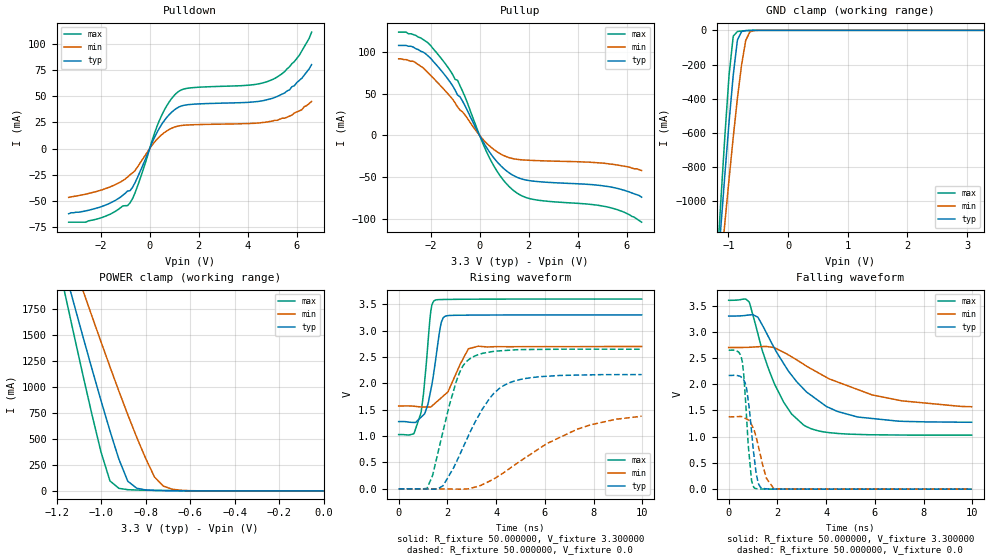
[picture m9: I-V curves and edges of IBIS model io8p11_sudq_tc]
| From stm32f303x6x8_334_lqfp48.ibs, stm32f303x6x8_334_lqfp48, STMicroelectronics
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|   Model io8p11_sudq_tc
[Model]  io8p11_sudq_tc
Model_type I/O
Polarity   Non-Inverting
Enable   Active-Low
Vinl =   0.990000V
Vinh =   2.310000V
Vmeas =  1.650000V
Cref =   30.000000pF
Rref =   100.000000M
Vref =   0.0V
C_comp   1.329900pF   1.255600pF   1.431200pF
[Temperature Range]   25.000000   0.125000k   -40.000000
[Pullup Reference]   3.300000V   2.700000V   3.600000V
[Pulldown Reference]   0.0V   0.0V   0.0V
[POWER Clamp Reference]   3.300000V   2.700000V   3.600000V
[GND Clamp Reference]   0.0V   0.0V   0.0V
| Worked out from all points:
|   slope of the pulldown table from 0 to 0.495 V, typ, clamps not added: 21.3 ohm
|   slope of the pullup table from 0 to 0.495 V, typ, clamps not added: 20.9 ohm
|   GND clamp passes 1 mA (typ) near -0.67 V on its own axis
|   POWER clamp passes 1 mA (typ) near -0.60 V on its own axis
|   rising waveform, R_fixture 50.000000, V_fixture 3.300000: 20-80 % time 415ps typ, 734ps min, 311ps max; typ from 1.27 V to 3.3 V
|   rising waveform, R_fixture 50.000000, V_fixture 0.0: 20-80 % time 1.47ns typ, 2.98ns min, 896ps max; typ from 0 V to 2.17 V
|   falling waveform, R_fixture 50.000000, V_fixture 3.300000: 20-80 % time 2.06ns typ, 3.13ns min, 1.29ns max; typ from 3.3 V to 1.27 V
|   falling waveform, R_fixture 50.000000, V_fixture 0.0: 20-80 % time 303ps typ, 447ps min, 236ps max; typ from 2.17 V to 0 V
[Pulldown]
|Voltage   I(typ)   I(min)   I(max)
-3.3V     -62mA      -46.4mA    -70mA
-2V       -55.5mA    -39.6mA    -66mA
-800mV    -40.04mA   -24.89mA   -51.58mA
-500mV    -27.57mA   -17.6mA    -36.07mA
400mV     19.71mA    11.36mA    27.01mA
700mV     29.83mA    16.93mA    40.97mA
1.1V      38.46mA    21.2mA     53.02mA
1.6V      41.98mA    22.62mA    57.7mA
4.1V      44.26mA    24mA       60.59mA
5V        47.9mA     26.3mA     65.8mA
5.9V      60mA       34mA       83mA
6.6V      80mA       45mA       111mA
[Pullup]
|Voltage   I(typ)   I(min)   I(max)
-3.3V     108mA      92mA       124mA
-2.7V     106mA      89mA       121mA
-2.2V     98mA       78.2mA     113mA
-1.4V     71.8mA     53.5mA     86.1mA
-900mV    48.51mA    34.23mA    66.14mA
-700mV    41.33mA    28.36mA    53.31mA
400mV     -19.77mA   -12.52mA   -26.8mA
900mV     -37.48mA   -22.89mA   -50.99mA
1.4V      -48.39mA   -28.06mA   -66.43mA
2.2V      -54.79mA   -29.98mA   -76.75mA
5.3V      -61.6mA    -34.2mA    -86.4mA
6.6V      -74mA      -42mA      -104mA
[GND_clamp]
|Voltage   I(typ)   I(min)   I(max)
-3.3V     -9.739A    -9.975A    -9.587A
-1.2V     -1.489A    -1.65A     -1.416A
-1.13V    -1.162A    -1.385A    -1.009A
-1.06V    -842.2mA   -1.125A    -616.9mA
-990mV    -537.1mA   -870.1mA   -263mA
-920mV    -262.4mA   -625.3mA   -33.96mA
-850mV    -56.94mA   -397.4mA   -7.08mA
-780mV    -7.011mA   -202.2mA   -3.71mA
-710mV    -1.778mA   -58.23mA   -1.736mA
-640mV    -550uA     -8.783mA   -542.4uA
-570mV    -109.8uA   -1.292mA   -86.89uA
3.28V     0A         0A         0A
[POWER_clamp]
|Voltage   I(typ)   I(min)   I(max)
-3.28V    9.897A     9.838A     9.594A
-1.16V    2.103A     2.419A     1.88A
-1.12V    1.788A     2.17A      1.488A
-1.08V    1.476A     1.923A     1.102A
-1V       868.1mA    1.435A     373.1mA
-960mV    578.2mA    1.196A     96.06mA
-880mV    93.24mA    734.1mA    12.01mA
-840mV    26.3mA     517.4mA    8.56mA
-760mV    5.106mA    134mA      5.119mA
-720mV    3.355mA    46.34mA    3.808mA
-600mV    1.005mA    2.564mA    1.072mA
0V        0A         0A         0A
[Ramp]
| variable   typ   min   max
dV/dt_r  1.30020/1.47318n   0.78894/2.97242n   1.58874/0.89490n
dV/dt_f  1.21380/2.06000n   0.65910/3.12889n   1.54248/1.29122n
R_load = 50.000000
[Rising Waveform]
R_fixture= 50.000000
V_fixture= 3.300000
V_fixture_min= 2.700000
V_fixture_max= 3.600000
|time   V(typ)   V(min)   V(max)
0s        1.275V     1.571V     1.03V
620.6ps   1.26V      1.567V     1.043V
920.9ps   1.36V      1.553V     1.452V
1.081ns   1.441V     1.553V     2.114V
1.321ns   1.881V     1.553V     3.378V
1.502ns   2.396V     1.627V     3.579V
1.702ns   3.049V     1.709V     3.59V
1.822ns   3.241V     1.758V     3.592V
2.863ns   3.295V     2.657V     3.597V
9.97ns    3.3V       2.7V       3.6V
[Rising Waveform]
R_fixture= 50.000000
V_fixture= 0.0
V_fixture_min= 0.0
V_fixture_max= 0.0
|time   V(typ)   V(min)   V(max)
0s        -62.44uV   -29.93uV   -44.66uV
1.161ns   -3.615mV   -95.42uV   9.224mV
1.401ns   -6.021mV   -580.1uV   271.7mV
1.822ns   59.25mV    -2.243mV   1.094V
2.362ns   504.1mV    -4.96mV    2.036V
3.003ns   1.144V     15.8mV     2.491V
3.884ns   1.8V       181.6mV    2.607V
4.725ns   2.041V     441.9mV    2.635V
7.307ns   2.157V     1.128V     2.649V
9.97ns    2.167V     1.378V     2.648V
[Falling Waveform]
R_fixture= 50.000000
V_fixture= 3.300000
V_fixture_min= 2.700000
V_fixture_max= 3.600000
|time   V(typ)   V(min)   V(max)
0s        3.3V       2.7V       3.6V
840.8ps   3.321V     2.704V     3.568V
1.201ns   3.276V     2.714V     2.957V
1.882ns   2.683V     2.697V     2.003V
2.583ns   2.172V     2.523V     1.432V
3.183ns   1.858V     2.349V     1.194V
4.024ns   1.573V     2.128V     1.083V
5.305ns   1.375V     1.897V     1.044V
7.107ns   1.294V     1.684V     1.032V
9.97ns    1.275V     1.571V     1.03V
[Falling Waveform]
R_fixture= 50.000000
V_fixture= 0.0
V_fixture_min= 0.0
V_fixture_max= 0.0
|time   V(typ)   V(min)   V(max)
0s        2.167V     1.378V     2.648V
400.4ps   2.16V      1.383V     2.616V
560.6ps   2.115V     1.376V     2.429V
740.7ps   1.903V     1.334V     1.322V
940.9ps   1.087V     1.226V     159.7mV
1.081ns   478.8mV    1.069V     16.4mV
1.301ns   38.87mV    652mV      3.318mV
1.542ns   6.531mV    219.5mV    1.906mV
1.862ns   2.279mV    5.862mV    1.343mV
9.97ns    -62.44uV   -29.93uV   -44.66uV
